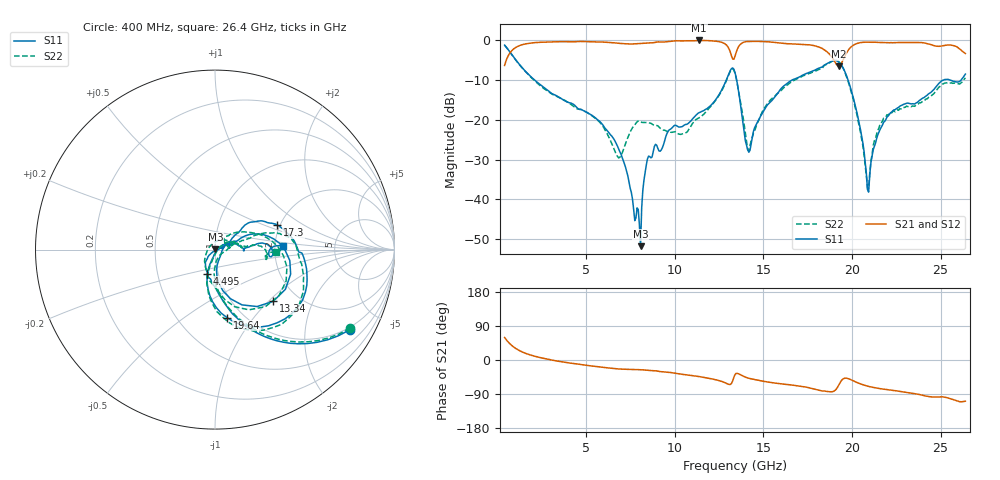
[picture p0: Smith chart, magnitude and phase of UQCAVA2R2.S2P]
!  Part Number  UQCAVA2R2
!  Description: RF capacitor  Mounting Orientation: Horizontal
!  Application:
# GHZ S DB R 50
! Freq  |S11|  S11 Ph  |S21|  S21 Ph  |S12|  S12 Ph  |S22|  S22 Ph
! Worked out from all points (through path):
!   401 points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, 400 MHz to 26.4 GHz, reference 50 ohm
!   highest |S21| = -0.01 dB at 11.38 GHz (marker M1); lowest = -6.5 dB at 19.25 GHz (marker M2)
!   group delay of S21, straight-line fit = 12.5 ps
!   lowest |S11| = -51.8 dB at 8.07 GHz (marker M3), VSWR 1.01, Z = 50.2 + j0.0714 ohm
!   |S11| at or under -10 dB: 2.1 GHz to 12.91 GHz (10.81 GHz wide, 144 % of centre); 13.49 GHz to 16.61 GHz (3.111 GHz wide, 20.7 % of centre); 19.78 GHz to 25.14 GHz (5.359 GHz wide, 23.9 % of centre)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
!   |S22| runs from -37.2 to -1.2 dB; largest |S21 - S12| = 0.0094
!   S11 on the Smith chart (normalised r, x): 400 MHz: 0.90, -3.40; 4.495 GHz: 0.89, -0.25; 13.34 GHz: 1.50, -1.07; 17.3 GHz: 1.93, +0.61; 19.64 GHz: 0.84, -0.75; 26.4 GHz: 2.20, +0.10
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0.4  -1.18 -30.9  -6.30 59.1  -6.34 59.2  -1.21 -30.2
1.635  -8.04 -72.5  -0.83 16.7  -0.87 16.8  -8.13 -72.1
4.495  -16.97 -107.3  -0.30 -10.3  -0.32 -10.1  -17.22 -106.3
4.755  -17.43 -108.4  -0.27 -12.3  -0.29 -12.1  -17.46 -108.2
6.835  -27.31 -136.1  -0.72 -23.7  -0.71 -23.4  -29.55 144.1
8.07  -51.76 16.0  -0.76 -25.7  -0.74 -25.3  -20.42 16.0
8.46  -29.80 30.5  -0.62 -27.2  -0.59 -26.8  -20.65 9.8
9.11  -27.79 10.1  -0.37 -30.1  -0.34 -29.7  -21.76 7.1
11.385  -18.15 22.1  -0.01 -43.7  -0.01 -43.6  -19.43 46.4
12.815  -10.93 16.9  -0.80 -59.5  -0.77 -59.5  -11.15 16.4
13.335  -7.25 -41.6  -4.73 -45.7  -4.70 -45.6  -7.45 -48.5
13.4  -8.08 -53.5  -4.00 -38.5  -3.97 -38.4  -8.29 -60.6
14.18  -28.13 -19.3  -0.28 -48.3  -0.24 -48.3  -27.73 -36.9
15.285  -15.98 35.7  -0.35 -58.4  -0.32 -58.5  -15.68 18.1
17.3  -8.58 21.6  -1.04 -70.6  -1.00 -70.7  -8.82 14.4
17.755  -7.74 13.8  -1.22 -75.2  -1.18 -75.4  -8.02 11.6
19.25  -5.43 -49.6  -6.49 -66.5  -6.45 -66.7  -5.32 -53.2
19.64  -8.30 -80.0  -3.60 -47.8  -3.56 -48.0  -8.50 -83.9
20.875  -37.49 -61.7  -0.44 -69.0  -0.41 -69.3  -37.14 -46.2
21.46  -23.73 23.0  -0.49 -74.7  -0.46 -75.0  -22.61 33.1
22.11  -18.61 15.5  -0.58 -79.0  -0.55 -79.3  -18.42 17.9
26.4  -8.48 3.1  -3.30 -108.6  -3.27 -109.1  -9.40 -1.9
